| IBIS file 144lqfp.ibs generated by Viper version: 2017.07.25
[IBIS Ver]   5.0
[Comment Char]   |_char
[File Name]   144lqfp.ibs
[File Rev]   1
[Date]   Wed Apr 18 11:55:22 2018
[Source]   Freescale Viper 2017.07.25
[Notes]
[Disclaimer] IMPORTANT NOTICE
  This information is provided on an AS IS basis and without warranty.
  IN NO EVENT SHALL Freescale BE LIABLE FOR INCIDENTAL OR CONSEQUENTIAL
  DAMAGES ARISING FROM USE OF THIS INFORMATION. THIS DISCLAIMER OF
  WARRANTY EXTENDS TO THE USER OF THE INFORMATION, AND TO THEIR CUSTOMERS
  OR USERS OF PRODUCTS  AND IS IN LIEU OF ALL WARRANTIES WHETHER EXPRESS,
  IMPLIED, OR STATUTORY, INCLUDING IMPLIED WARRANTIES OF MERCHANTABILITY
  OR FITNESS FOR PARTICULAR PURPOSE.
  Freescale does not represent or warrant that the information furnished
  hereunder is free of infringement of any third party patents,
  copyrights, trade secrets, or other intellectual property rights.
  Freescale does not represent or warrant that the information is free of
  defect, or that it meets any particular standard, requirements or need
  of the user of the infomation or their customers.
  Freescale reserves the right to change the information in this file
  without notice.
   http://www.freescale.com
[Copyright]   (C) Copyright Freescale 2004 - 2018, All Rights Reserved.
|   144LQFP
[Component]   144LQFP
[Manufacturer]   FREESCALE
[Package]
| variable   typ   min   max
R_pkg   0.23631   0.21255   0.27668
L_pkg   6.725e-09   6.219e-09   7.763e-09
C_pkg   7.045e-13   5.974e-13   8.478e-13
[Pin] signal_name   model_name   R_pin   L_pin   C_pin
1   GPIO_EMC_14   gpio   0.27319   7.763e-09 7.620e-13
2   GPIO_EMC_13   gpio   0.24922   7.284e-09 7.877e-13
3   GPIO_EMC_12   gpio   0.25596   7.201e-09 8.198e-13
4   GPIO_EMC_11   gpio   0.24258   6.690e-09 7.773e-13
5   VDD_SOC_IN   POWER   NA   NA   NA
6   NC   NC   NA   NA   NA
7   GPIO_EMC_10   gpio   0.22716   6.478e-09 7.216e-13
8   GPIO_EMC_09   gpio   0.23253   6.549e-09 7.118e-13
9   GPIO_EMC_08   gpio   0.21792   6.312e-09 7.130e-13
10   GPIO_EMC_07   gpio   0.22722   6.434e-09 6.632e-13
11   NVCC_GPIO   POWER   NA   NA   NA
12   GPIO_EMC_06   gpio   0.21323   6.350e-09 6.818e-13
13   GPIO_EMC_05   gpio   0.2234   6.650e-09 6.747e-13
14   GPIO_EMC_04   gpio   0.22404   6.772e-09 6.509e-13
15   GPIO_EMC_03   gpio   0.21613   6.689e-09 6.468e-13
16   GPIO_EMC_02   gpio   0.22926   6.931e-09 6.556e-13
17   GPIO_EMC_01   gpio   0.22816   6.913e-09 6.110e-13
18   GPIO_EMC_00   gpio   0.26205   7.440e-09 6.211e-13
19   GPIO_SD_B1_11   gpio   0.26047   7.181e-09 6.075e-13
20   NVCC_GPIO   POWER   NA   NA   NA
21   GPIO_SD_B1_10   gpio   0.24307   6.886e-09 6.379e-13
22   GPIO_SD_B1_09   gpio   0.23465   6.862e-09 6.668e-13
23   GPIO_SD_B1_08   gpio   0.22372   6.608e-09 6.606e-13
24   GPIO_SD_B1_07   gpio   0.23361   6.711e-09 6.776e-13
25   GPIO_SD_B1_06   gpio   0.22833   6.612e-09 6.719e-13
26   GPIO_SD_B1_05   gpio   0.24019   6.758e-09 7.358e-13
27   GPIO_SD_B1_04   gpio   0.23557   6.606e-09 7.328e-13
28   GPIO_SD_B1_03   gpio   0.25289   6.532e-09 7.645e-13
29   NVCC_GPIO   POWER   NA   NA   NA
30   GPIO_SD_B1_02   gpio   0.26218   6.601e-09 7.491e-13
31   VDD_SOC_IN   POWER   NA   NA   NA
32   GPIO_SD_B1_01   gpio   0.25369   6.647e-09 8.100e-13
33   GPIO_SD_B1_00   gpio   0.27668   6.878e-09 8.292e-13
34   DCDC_IN   POWER   NA   NA   NA
35   DCDC_GND   GND   NA   NA   NA
36   NC   NC   NA   NA   NA
37   DCDC_PSWITCH   POWER   NA   NA   NA
38   DCDC_IN_Q   POWER   NA   NA   NA
39   VDD_SOC_IN   POWER   NA   NA   NA
40   NC   NC   NA   NA   NA
41   GPIO_SD_B0_06   gpio   0.24784   6.847e-09 7.446e-13
42   GPIO_SD_B0_05   gpio   0.23425   6.606e-09 7.288e-13
43   GPIO_SD_B0_04   gpio   0.23978   6.581e-09 7.445e-13
44   NVCC_SD0   POWER   NA   NA   NA
45   GPIO_SD_B0_03   gpio   0.23499   6.428e-09 7.074e-13
46   GPIO_SD_B0_02   gpio   0.22524   6.518e-09 6.811e-13
47   GPIO_SD_B0_01   gpio   0.21255   6.369e-09 6.751e-13
48   GPIO_SD_B0_00   gpio   0.22018   6.545e-09 6.743e-13
49   ONOFF   gpio   0.22022   6.591e-09 6.545e-13
50   POR_B   gpio   0.22145   6.657e-09 6.500e-13
51   TEST_MODE   gpio   0.21301   6.530e-09 6.305e-13
52   WAKEUP   gpio   0.22627   6.774e-09 6.197e-13
53   PMIC_ON_REQ   gpio   0.22495   6.778e-09 6.119e-13
54   PMIC_STBY_REQ   gpio   0.25873   7.238e-09 6.013e-13
55   VDD_SNVS_IN   POWER   NA   NA   NA
56   VDD_SNVS_CAP   POWER   NA   NA   NA
57   RTC_XTALI   NC   0.23318   6.569e-09 6.200e-13
58   RTC_XTALO   NC   0.22932   6.412e-09 6.458e-13
59   USB_OTG1_VBUS   NC   NA   NA   NA
60   NC   NC   NA   NA   NA
61   VDD_USB_CAP   NC   NA   NA   NA
62   USB_OTG1_DN   NC   0.23049   6.219e-09 6.692e-13
63   USB_OTG1_DP   NC   0.23382   6.238e-09 7.381e-13
64   NGND_KEL0   GND   NA   NA   NA
65   VDD_HIGH_CAP   POWER   NA   NA   NA
66   USB_OTG1_CHD_B   NC   0.23453   6.262e-09 7.522e-13
67   XTALI   NC   0.24304   6.614e-09 7.504e-13
68   XTALO   NC   0.25011   6.724e-09 7.704e-13
69   VDD_HIGH_IN   POWER   NA   NA   NA
70   NC   NC   NA   NA   NA
71   GPANAIO   NC   0.25746   6.958e-09 7.980e-13
72   NVCC_PLL   POWER   NA   NA   NA
73   VDDA_ADC_3P3   POWER   NA   NA   NA
74   GPIO_AD_B1_15   gpio   0.25409   6.952e-09 8.420e-13
75   GPIO_AD_B1_14   gpio   0.25632   6.963e-09 8.478e-13
76   GPIO_AD_B1_13   gpio   0.25252   6.929e-09 7.716e-13
77   NC   NC   NA   NA   NA
78   GPIO_AD_B1_12   gpio   0.24265   6.738e-09 7.369e-13
79   GPIO_AD_B1_11   gpio   0.23034   6.449e-09 7.323e-13
80   GPIO_AD_B1_10   gpio   0.23308   6.558e-09 7.263e-13
81   GPIO_AD_B1_09   gpio   0.22922   6.558e-09 7.224e-13
82   GPIO_AD_B1_08   gpio   0.21958   6.371e-09 7.084e-13
83   GPIO_AD_B1_07   gpio   0.2282   6.393e-09 7.151e-13
84   GPIO_AD_B1_06   gpio   0.23128   6.391e-09 6.709e-13
85   NC   NC   NA   NA   NA
86   VDD_SOC_IN   POWER   NA   NA   NA
87   GPIO_AD_B1_05   gpio   0.22109   6.396e-09 6.938e-13
88   GPIO_AD_B1_04   gpio   0.23176   6.820e-09 6.617e-13
89   GPIO_AD_B1_03   gpio   0.2259   6.807e-09 6.341e-13
90   GPIO_AD_B1_02   gpio   0.2578   7.521e-09 5.976e-13
91   GPIO_AD_B1_01   gpio   0.24916   7.279e-09 5.978e-13
92   GPIO_AD_B1_00   gpio   0.24244   6.931e-09 6.196e-13
93   GPIO_AD_B0_15   gpio   0.23462   6.875e-09 6.702e-13
94   GPIO_AD_B0_14   gpio   0.21942   6.541e-09 6.321e-13
95   GPIO_AD_B0_13   gpio   0.22448   6.708e-09 6.624e-13
96   GPIO_AD_B0_12   gpio   0.22263   6.609e-09 6.816e-13
97   GPIO_AD_B0_11   gpio   0.21559   6.396e-09 6.793e-13
98   GPIO_AD_B0_10   gpio   0.22709   6.461e-09 6.804e-13
99   GPIO_AD_B0_09   gpio   0.22347   6.302e-09 7.026e-13
100   GPIO_AD_B0_08   gpio   0.23203   6.436e-09 7.127e-13
101   GPIO_AD_B0_07   gpio   0.2232   6.229e-09 7.231e-13
102   VDD_SOC_IN   POWER   NA   NA   NA
103   NC   NC   NA   NA   NA
104   NC   NC   NA   NA   NA
105   GPIO_AD_B0_06   gpio   0.23499   6.864e-09 7.362e-13
106   GPIO_AD_B0_05   gpio   0.24648   7.161e-09 8.049e-13
107   GPIO_AD_B0_04   gpio   0.24526   7.309e-09 8.157e-13
108   GPIO_AD_B0_03   gpio   0.26036   7.662e-09 7.794e-13
109   GPIO_AD_B0_02   gpio   0.26315   7.383e-09 7.807e-13
110   GPIO_AD_B0_01   gpio   0.26589   7.252e-09 8.095e-13
111   GPIO_AD_B0_00   gpio   0.26336   6.854e-09 7.971e-13
112   NC   NC   NA   NA   NA
113   NC   NC   NA   NA   NA
114   VDD_SOC_IN   POWER   NA   NA   NA
115   GPIO_EMC_41   gpio   0.22452   6.470e-09 7.317e-13
116   GPIO_EMC_40   gpio   0.23083   6.535e-09 7.263e-13
117   GPIO_EMC_39   gpio   0.22168   6.332e-09 7.381e-13
118   GPIO_EMC_38   gpio   0.23093   6.497e-09 7.401e-13
119   GPIO_EMC_37   gpio   0.23081   6.423e-09 7.303e-13
120   GPIO_EMC_36   gpio   0.22714   6.494e-09 7.167e-13
121   GPIO_EMC_35   gpio   0.21462   6.464e-09 6.823e-13
122   GPIO_EMC_34   gpio   0.22438   6.655e-09 6.932e-13
123   GPIO_EMC_33   gpio   0.21793   6.470e-09 6.273e-13
124   GPIO_EMC_32   gpio   0.23516   6.805e-09 6.307e-13
125   GPIO_EMC_31   gpio   0.24148   6.948e-09 6.305e-13
126   GPIO_EMC_30   gpio   0.25496   7.362e-09 6.088e-13
127   GPIO_EMC_29   gpio   0.2576   7.422e-09 5.974e-13
128   GPIO_EMC_28   gpio   0.24014   7.035e-09 6.374e-13
129   GPIO_EMC_27   gpio   0.22626   6.621e-09 6.383e-13
130   GPIO_EMC_26   gpio   0.23483   6.649e-09 6.554e-13
131   GPIO_EMC_25   gpio   0.23202   6.549e-09 6.551e-13
132   GPIO_EMC_24   gpio   0.22925   6.491e-09 6.599e-13
133   GPIO_EMC_23   gpio   0.2212   6.232e-09 6.790e-13
134   VDD_SOC_IN   POWER   NA   NA   NA
135   NC   NC   NA   NA   NA
136   GPIO_EMC_22   gpio   0.22481   6.353e-09 6.683e-13
137   GPIO_EMC_21   gpio   0.22739   6.524e-09 7.340e-13
138   GPIO_EMC_20   gpio   0.24177   6.765e-09 7.486e-13
139   GPIO_EMC_19   gpio   0.23809   6.755e-09 7.541e-13
140   GPIO_EMC_18   gpio   0.24061   6.892e-09 7.906e-13
141   GPIO_EMC_17   gpio   0.23882   6.883e-09 8.027e-13
142   GPIO_EMC_16   gpio   0.25453   7.072e-09 8.171e-13
143   GPIO_EMC_15   gpio   0.257   7.017e-09 8.337e-13
144   NC   NC   NA   NA   NA
145   NC   NC   NA   NA   NA
[Pin Mapping]   pulldown_ref   pullup_ref
1   NC   NC
2   NC   NC
3   NC   NC
4   NC   NC
5   NC   VDD_SOC_IN
6   NC   NC
7   NC   NC
8   NC   NC
9   NC   NC
10   NC   NC
11   NC   NVCC_GPIO
12   NC   NC
13   NC   NC
14   NC   NC
15   NC   NC
16   NC   NC
17   NC   NC
18   NC   NC
19   NC   NC
20   NC   NVCC_GPIO
21   NC   NC
22   NC   NC
23   NC   NC
24   NC   NC
25   NC   NC
26   NC   NC
27   NC   NC
28   NC   NC
29   NC   NVCC_GPIO
30   NC   NC
31   NC   VDD_SOC_IN
32   NC   NC
33   NC   NC
34   NC   DCDC_IN
35   DCDC_GND   NC
36   NC   NC
37   NC   DCDC_PSWITCH
38   NC   DCDC_IN_Q
39   NC   VDD_SOC_IN
40   NC   NC
41   NC   NC
42   NC   NC
43   NC   NC
44   NC   NVCC_SD0
45   NC   NC
46   NC   NC
47   NC   NC
48   NC   NC
49   NC   NC
50   NC   NC
51   NC   NC
52   NC   NC
53   NC   NC
54   NC   NC
55   NC   VDD_SNVS_IN
56   NC   VDD_SNVS_CAP
57   NC   NC
58   NC   NC
59   NC   NC
60   NC   NC
61   NC   NC
62   NC   NC
63   NC   NC
64   NGND_KEL0   NC
65   NC   VDD_HIGH_CAP
66   NC   NC
67   NC   NC
68   NC   NC
69   NC   VDD_HIGH_IN
70   NC   NC
71   NC   NC
72   NC   NVCC_PLL
73   NC   VDDA_ADC_3P3
74   NC   NC
75   NC   NC
76   NC   NC
77   NC   NC
78   NC   NC
79   NC   NC
80   NC   NC
81   NC   NC
82   NC   NC
83   NC   NC
84   NC   NC
85   NC   NC
86   NC   VDD_SOC_IN
87   NC   NC
88   NC   NC
89   NC   NC
90   NC   NC
91   NC   NC
92   NC   NC
93   NC   NC
94   NC   NC
95   NC   NC
96   NC   NC
97   NC   NC
98   NC   NC
99   NC   NC
100   NC   NC
101   NC   NC
102   NC   VDD_SOC_IN
103   NC   NC
104   NC   NC
105   NC   NC
106   NC   NC
107   NC   NC
108   NC   NC
109   NC   NC
110   NC   NC
111   NC   NC
112   NC   NC
113   NC   NC
114   NC   VDD_SOC_IN
115   NC   NC
116   NC   NC
117   NC   NC
118   NC   NC
119   NC   NC
120   NC   NC
121   NC   NC
122   NC   NC
123   NC   NC
124   NC   NC
125   NC   NC
126   NC   NC
127   NC   NC
128   NC   NC
129   NC   NC
130   NC   NC
131   NC   NC
132   NC   NC
133   NC   NC
134   NC   VDD_SOC_IN
135   NC   NC
136   NC   NC
137   NC   NC
138   NC   NC
139   NC   NC
140   NC   NC
141   NC   NC
142   NC   NC
143   NC   NC
144   NC   NC
145   NC   NC
|*   Model Selector   *
[Model Selector] gpio
gpio1p8_ds111_sr111_mio   GPIO, 1.8V,extra drive,fast sr,max fsel
gpio1p8_ds111_sr110_mio   GPIO, 1.8V,extra drive,fast sr,fast fsel
gpio1p8_ds111_sr101_mio   GPIO, 1.8V,extra drive,fast sr,medium fsel
gpio1p8_ds111_sr100_mio   GPIO, 1.8V,extra drive,fast sr,slow fsel
gpio1p8_ds111_sr011_mio   GPIO, 1.8V,extra drive,slow sr,max fsel
gpio1p8_ds111_sr010_mio   GPIO, 1.8V,extra drive,slow sr,fast fsel
gpio1p8_ds111_sr001_mio   GPIO, 1.8V,extra drive,slow sr,medium fsel
gpio1p8_ds111_sr000_mio   GPIO, 1.8V,extra drive,slow sr,slow fsel
gpio1p8_ds110_sr111_mio   GPIO, 1.8V,extra drive,fast sr,max fsel
gpio1p8_ds110_sr110_mio   GPIO, 1.8V,extra drive,fast sr,fast fsel
gpio1p8_ds110_sr101_mio   GPIO, 1.8V,extra drive,fast sr,medium fsel
gpio1p8_ds110_sr100_mio   GPIO, 1.8V,extra drive,fast sr,slow fsel
gpio1p8_ds110_sr011_mio   GPIO, 1.8V,extra drive,slow sr,max fsel
gpio1p8_ds110_sr010_mio   GPIO, 1.8V,extra drive,slow sr,fast fsel
gpio1p8_ds110_sr001_mio   GPIO, 1.8V,extra drive,slow sr,medium fsel
gpio1p8_ds110_sr000_mio   GPIO, 1.8V,extra drive,slow sr,slow fsel
gpio1p8_ds101_sr111_mio   GPIO, 1.8V,max drive,fast sr,max fsel
gpio1p8_ds101_sr110_mio   GPIO, 1.8V,max drive,fast sr,fast fsel
gpio1p8_ds101_sr101_mio   GPIO, 1.8V,max drive,fast sr,medium fsel
gpio1p8_ds101_sr100_mio   GPIO, 1.8V,max drive,fast sr,slow fsel
gpio1p8_ds101_sr011_mio   GPIO, 1.8V,max drive,slow sr,max fsel
gpio1p8_ds101_sr010_mio   GPIO, 1.8V,max drive,slow sr,fast fsel
gpio1p8_ds101_sr001_mio   GPIO, 1.8V,max drive,slow sr,medium fsel
gpio1p8_ds101_sr000_mio   GPIO, 1.8V,max drive,slow sr,slow fsel
gpio1p8_ds100_sr111_mio   GPIO, 1.8V,extra drive,fast sr,max fsel
gpio1p8_ds100_sr110_mio   GPIO, 1.8V,extra drive,fast sr,fast fsel
gpio1p8_ds100_sr101_mio   GPIO, 1.8V,extra drive,fast sr,medium fsel
gpio1p8_ds100_sr100_mio   GPIO, 1.8V,extra drive,fast sr,slow fsel
gpio1p8_ds100_sr011_mio   GPIO, 1.8V,extra drive,slow sr,max fsel
gpio1p8_ds100_sr010_mio   GPIO, 1.8V,extra drive,slow sr,fast fsel
gpio1p8_ds100_sr001_mio   GPIO, 1.8V,extra drive,slow sr,medium fsel
gpio1p8_ds100_sr000_mio   GPIO, 1.8V,extra drive,slow sr,slow fsel
gpio1p8_ds011_sr111_mio   GPIO, 1.8V,high drive,fast sr,max fsel
gpio1p8_ds011_sr110_mio   GPIO, 1.8V,high drive,fast sr,fast fsel
gpio1p8_ds011_sr101_mio   GPIO, 1.8V,high drive,fast sr,medium fsel
gpio1p8_ds011_sr100_mio   GPIO, 1.8V,high drive,fast sr,slow fsel
gpio1p8_ds011_sr011_mio   GPIO, 1.8V,high drive,slow sr,max fsel
gpio1p8_ds011_sr010_mio   GPIO, 1.8V,high drive,slow sr,fast fsel
gpio1p8_ds011_sr001_mio   GPIO, 1.8V,high drive,slow sr,medium fsel
gpio1p8_ds011_sr000_mio   GPIO, 1.8V,high drive,slow sr,slow fsel
gpio1p8_ds010_sr111_mio   GPIO, 1.8V,medium drive,fast sr,max fsel
gpio1p8_ds010_sr110_mio   GPIO, 1.8V,medium drive,fast sr,fast fsel
gpio1p8_ds010_sr101_mio   GPIO, 1.8V,medium drive,fast sr,medium fsel
gpio1p8_ds010_sr100_mio   GPIO, 1.8V,medium drive,fast sr,slow fsel
gpio1p8_ds010_sr011_mio   GPIO, 1.8V,medium drive,slow sr,max fsel
gpio1p8_ds010_sr010_mio   GPIO, 1.8V,medium drive,slow sr,fast fsel
gpio1p8_ds010_sr001_mio   GPIO, 1.8V,medium drive,slow sr,medium fsel
gpio1p8_ds010_sr000_mio   GPIO, 1.8V,medium drive,slow sr,slow fsel
gpio1p8_ds001_sr111_mio   GPIO, 1.8V,low drive,fast sr,max fsel
gpio1p8_ds001_sr110_mio   GPIO, 1.8V,low drive,fast sr,fast fsel
gpio1p8_ds001_sr101_mio   GPIO, 1.8V,low drive,fast sr,medium fsel
gpio1p8_ds001_sr100_mio   GPIO, 1.8V,low drive,fast sr,slow fsel
gpio1p8_ds001_sr011_mio   GPIO, 1.8V,low drive,slow sr,max fsel
gpio1p8_ds001_sr010_mio   GPIO, 1.8V,low drive,slow sr,fast fsel
gpio1p8_ds001_sr001_mio   GPIO, 1.8V,low drive,slow sr,medium fsel
gpio1p8_ds001_sr000_mio   GPIO, 1.8V,low drive,slow sr,slow fsel
gpio2p5_ds111_sr111_mio   GPIO, 2.5V,extra drive,fast sr,max fsel
gpio2p5_ds111_sr110_mio   GPIO, 2.5V,extra drive,fast sr,fast fsel
gpio2p5_ds111_sr101_mio   GPIO, 2.5V,extra drive,fast sr,medium fsel
gpio2p5_ds111_sr100_mio   GPIO, 2.5V,extra drive,fast sr,slow fsel
gpio2p5_ds111_sr011_mio   GPIO, 2.5V,extra drive,slow sr,max fsel
gpio2p5_ds111_sr010_mio   GPIO, 2.5V,extra drive,slow sr,fast fsel
gpio2p5_ds111_sr001_mio   GPIO, 2.5V,extra drive,slow sr,medium fsel
gpio2p5_ds111_sr000_mio   GPIO, 2.5V,extra drive,slow sr,slow fsel
gpio2p5_ds110_sr111_mio   GPIO, 2.5V,extra drive,fast sr,max fsel
gpio2p5_ds110_sr110_mio   GPIO, 2.5V,extra drive,fast sr,fast fsel
gpio2p5_ds110_sr101_mio   GPIO, 2.5V,extra drive,fast sr,medium fsel
gpio2p5_ds110_sr100_mio   GPIO, 2.5V,extra drive,fast sr,slow fsel
gpio2p5_ds110_sr011_mio   GPIO, 2.5V,extra drive,slow sr,max fsel
gpio2p5_ds110_sr010_mio   GPIO, 2.5V,extra drive,slow sr,fast fsel
gpio2p5_ds110_sr001_mio   GPIO, 2.5V,extra drive,slow sr,medium fsel
gpio2p5_ds110_sr000_mio   GPIO, 2.5V,extra drive,slow sr,slow fsel
gpio2p5_ds101_sr111_mio   GPIO, 2.5V,max drive,fast sr,max fsel
gpio2p5_ds101_sr110_mio   GPIO, 2.5V,max drive,fast sr,fast fsel
gpio2p5_ds101_sr101_mio   GPIO, 2.5V,max drive,fast sr,medium fsel
gpio2p5_ds101_sr100_mio   GPIO, 2.5V,max drive,fast sr,slow fsel
gpio2p5_ds101_sr011_mio   GPIO, 2.5V,max drive,slow sr,max fsel
gpio2p5_ds101_sr010_mio   GPIO, 2.5V,max drive,slow sr,fast fsel
gpio2p5_ds101_sr001_mio   GPIO, 2.5V,max drive,slow sr,medium fsel
gpio2p5_ds101_sr000_mio   GPIO, 2.5V,max drive,slow sr,slow fsel
gpio2p5_ds100_sr111_mio   GPIO, 2.5V,extra drive,fast sr,max fsel
gpio2p5_ds100_sr110_mio   GPIO, 2.5V,extra drive,fast sr,fast fsel
gpio2p5_ds100_sr101_mio   GPIO, 2.5V,extra drive,fast sr,medium fsel
gpio2p5_ds100_sr100_mio   GPIO, 2.5V,extra drive,fast sr,slow fsel
gpio2p5_ds100_sr011_mio   GPIO, 2.5V,extra drive,slow sr,max fsel
gpio2p5_ds100_sr010_mio   GPIO, 2.5V,extra drive,slow sr,fast fsel
gpio2p5_ds100_sr001_mio   GPIO, 2.5V,extra drive,slow sr,medium fsel
gpio2p5_ds100_sr000_mio   GPIO, 2.5V,extra drive,slow sr,slow fsel
gpio2p5_ds011_sr111_mio   GPIO, 2.5V,high drive,fast sr,max fsel
gpio2p5_ds011_sr110_mio   GPIO, 2.5V,high drive,fast sr,fast fsel
gpio2p5_ds011_sr101_mio   GPIO, 2.5V,high drive,fast sr,medium fsel
gpio2p5_ds011_sr100_mio   GPIO, 2.5V,high drive,fast sr,slow fsel
gpio2p5_ds011_sr011_mio   GPIO, 2.5V,high drive,slow sr,max fsel
gpio2p5_ds011_sr010_mio   GPIO, 2.5V,high drive,slow sr,fast fsel
gpio2p5_ds011_sr001_mio   GPIO, 2.5V,high drive,slow sr,medium fsel
gpio2p5_ds011_sr000_mio   GPIO, 2.5V,high drive,slow sr,slow fsel
gpio2p5_ds010_sr111_mio   GPIO, 2.5V,medium drive,fast sr,max fsel
gpio2p5_ds010_sr110_mio   GPIO, 2.5V,medium drive,fast sr,fast fsel
gpio2p5_ds010_sr101_mio   GPIO, 2.5V,medium drive,fast sr,medium fsel
gpio2p5_ds010_sr100_mio   GPIO, 2.5V,medium drive,fast sr,slow fsel
gpio2p5_ds010_sr011_mio   GPIO, 2.5V,medium drive,slow sr,max fsel
gpio2p5_ds010_sr010_mio   GPIO, 2.5V,medium drive,slow sr,fast fsel
gpio2p5_ds010_sr001_mio   GPIO, 2.5V,medium drive,slow sr,medium fsel
gpio2p5_ds010_sr000_mio   GPIO, 2.5V,medium drive,slow sr,slow fsel
gpio2p5_ds001_sr111_mio   GPIO, 2.5V,low drive,fast sr,max fsel
gpio2p5_ds001_sr110_mio   GPIO, 2.5V,low drive,fast sr,fast fsel
gpio2p5_ds001_sr101_mio   GPIO, 2.5V,low drive,fast sr,medium fsel
gpio2p5_ds001_sr100_mio   GPIO, 2.5V,low drive,fast sr,slow fsel
gpio2p5_ds001_sr011_mio   GPIO, 2.5V,low drive,slow sr,max fsel
gpio2p5_ds001_sr010_mio   GPIO, 2.5V,low drive,slow sr,fast fsel
gpio2p5_ds001_sr001_mio   GPIO, 2.5V,low drive,slow sr,medium fsel
gpio2p5_ds001_sr000_mio   GPIO, 2.5V,low drive,slow sr,slow fsel
gpio3p3_ds111_sr111_mio   GPIO, 3.3V,extra drive,fast sr,max fsel
gpio3p3_ds111_sr110_mio   GPIO, 3.3V,extra drive,fast sr,fast fsel
gpio3p3_ds111_sr101_mio   GPIO, 3.3V,extra drive,fast sr,medium fsel
gpio3p3_ds111_sr100_mio   GPIO, 3.3V,extra drive,fast sr,slow fsel
gpio3p3_ds111_sr011_mio   GPIO, 3.3V,extra drive,slow sr,max fsel
gpio3p3_ds111_sr010_mio   GPIO, 3.3V,extra drive,slow sr,fast fsel
gpio3p3_ds111_sr001_mio   GPIO, 3.3V,extra drive,slow sr,medium fsel
gpio3p3_ds111_sr000_mio   GPIO, 3.3V,extra drive,slow sr,slow fsel
gpio3p3_ds110_sr111_mio   GPIO, 3.3V,extra drive,fast sr,max fsel
gpio3p3_ds110_sr110_mio   GPIO, 3.3V,extra drive,fast sr,fast fsel
gpio3p3_ds110_sr101_mio   GPIO, 3.3V,extra drive,fast sr,medium fsel
gpio3p3_ds110_sr100_mio   GPIO, 3.3V,extra drive,fast sr,slow fsel
gpio3p3_ds110_sr011_mio   GPIO, 3.3V,extra drive,slow sr,max fsel
gpio3p3_ds110_sr010_mio   GPIO, 3.3V,extra drive,slow sr,fast fsel
gpio3p3_ds110_sr001_mio   GPIO, 3.3V,extra drive,slow sr,medium fsel
gpio3p3_ds110_sr000_mio   GPIO, 3.3V,extra drive,slow sr,slow fsel
gpio3p3_ds101_sr111_mio   GPIO, 3.3V,max drive,fast sr,max fsel
gpio3p3_ds101_sr110_mio   GPIO, 3.3V,max drive,fast sr,fast fsel
gpio3p3_ds101_sr101_mio   GPIO, 3.3V,max drive,fast sr,medium fsel
gpio3p3_ds101_sr100_mio   GPIO, 3.3V,max drive,fast sr,slow fsel
gpio3p3_ds101_sr011_mio   GPIO, 3.3V,max drive,slow sr,max fsel
gpio3p3_ds101_sr010_mio   GPIO, 3.3V,max drive,slow sr,fast fsel
gpio3p3_ds101_sr001_mio   GPIO, 3.3V,max drive,slow sr,medium fsel
gpio3p3_ds101_sr000_mio   GPIO, 3.3V,max drive,slow sr,slow fsel
gpio3p3_ds100_sr111_mio   GPIO, 3.3V,extra drive,fast sr,max fsel
gpio3p3_ds100_sr110_mio   GPIO, 3.3V,extra drive,fast sr,fast fsel
gpio3p3_ds100_sr101_mio   GPIO, 3.3V,extra drive,fast sr,medium fsel
gpio3p3_ds100_sr100_mio   GPIO, 3.3V,extra drive,fast sr,slow fsel
gpio3p3_ds100_sr011_mio   GPIO, 3.3V,extra drive,slow sr,max fsel
gpio3p3_ds100_sr010_mio   GPIO, 3.3V,extra drive,slow sr,fast fsel
gpio3p3_ds100_sr001_mio   GPIO, 3.3V,extra drive,slow sr,medium fsel
gpio3p3_ds100_sr000_mio   GPIO, 3.3V,extra drive,slow sr,slow fsel
gpio3p3_ds011_sr111_mio   GPIO, 3.3V,high drive,fast sr,max fsel
gpio3p3_ds011_sr110_mio   GPIO, 3.3V,high drive,fast sr,fast fsel
gpio3p3_ds011_sr101_mio   GPIO, 3.3V,high drive,fast sr,medium fsel
gpio3p3_ds011_sr100_mio   GPIO, 3.3V,high drive,fast sr,slow fsel
gpio3p3_ds011_sr011_mio   GPIO, 3.3V,high drive,slow sr,max fsel
gpio3p3_ds011_sr010_mio   GPIO, 3.3V,high drive,slow sr,fast fsel
gpio3p3_ds011_sr001_mio   GPIO, 3.3V,high drive,slow sr,medium fsel
gpio3p3_ds011_sr000_mio   GPIO, 3.3V,high drive,slow sr,slow fsel
gpio3p3_ds010_sr111_mio   GPIO, 3.3V,medium drive,fast sr,max fsel
gpio3p3_ds010_sr110_mio   GPIO, 3.3V,medium drive,fast sr,fast fsel
gpio3p3_ds010_sr101_mio   GPIO, 3.3V,medium drive,fast sr,medium fsel
gpio3p3_ds010_sr100_mio   GPIO, 3.3V,medium drive,fast sr,slow fsel
gpio3p3_ds010_sr011_mio   GPIO, 3.3V,medium drive,slow sr,max fsel
gpio3p3_ds010_sr010_mio   GPIO, 3.3V,medium drive,slow sr,fast fsel
gpio3p3_ds010_sr001_mio   GPIO, 3.3V,medium drive,slow sr,medium fsel
gpio3p3_ds010_sr000_mio   GPIO, 3.3V,medium drive,slow sr,slow fsel
gpio3p3_ds001_sr111_mio   GPIO, 3.3V,low drive,fast sr,max fsel
gpio3p3_ds001_sr110_mio   GPIO, 3.3V,low drive,fast sr,fast fsel
gpio3p3_ds001_sr101_mio   GPIO, 3.3V,low drive,fast sr,medium fsel
gpio3p3_ds001_sr100_mio   GPIO, 3.3V,low drive,fast sr,slow fsel
gpio3p3_ds001_sr011_mio   GPIO, 3.3V,low drive,slow sr,max fsel
gpio3p3_ds001_sr010_mio   GPIO, 3.3V,low drive,slow sr,fast fsel
gpio3p3_ds001_sr001_mio   GPIO, 3.3V,low drive,slow sr,medium fsel
gpio3p3_ds001_sr000_mio   GPIO, 3.3V,low drive,slow sr,slow fsel
| End [Component] 144LQFP
| Models and submodels in the file (168): gpio1p8_ds001_sr000_mio (I/O), gpio1p8_ds001_sr001_mio (I/O), gpio1p8_ds001_sr010_mio (I/O), gpio1p8_ds001_sr011_mio (I/O), gpio1p8_ds001_sr100_mio (I/O), gpio1p8_ds001_sr101_mio (I/O), gpio1p8_ds001_sr110_mio (I/O), gpio1p8_ds001_sr111_mio (I/O), gpio1p8_ds010_sr000_mio (I/O), gpio1p8_ds010_sr001_mio (I/O), gpio1p8_ds010_sr010_mio (I/O), gpio1p8_ds010_sr011_mio (I/O), gpio1p8_ds010_sr100_mio (I/O), gpio1p8_ds010_sr101_mio (I/O), gpio1p8_ds010_sr110_mio (I/O), gpio1p8_ds010_sr111_mio (I/O), gpio1p8_ds011_sr000_mio (I/O), gpio1p8_ds011_sr001_mio (I/O), gpio1p8_ds011_sr010_mio (I/O), gpio1p8_ds011_sr011_mio (I/O), gpio1p8_ds011_sr100_mio (I/O), gpio1p8_ds011_sr101_mio (I/O), gpio1p8_ds011_sr110_mio (I/O), gpio1p8_ds011_sr111_mio (I/O), gpio1p8_ds100_sr000_mio (I/O), gpio1p8_ds100_sr001_mio (I/O), gpio1p8_ds100_sr010_mio (I/O), gpio1p8_ds100_sr011_mio (I/O), gpio1p8_ds100_sr100_mio (I/O), gpio1p8_ds100_sr101_mio (I/O), gpio1p8_ds100_sr110_mio (I/O), gpio1p8_ds100_sr111_mio (I/O), gpio1p8_ds101_sr000_mio (I/O), gpio1p8_ds101_sr001_mio (I/O), gpio1p8_ds101_sr010_mio (I/O), gpio1p8_ds101_sr011_mio (I/O), gpio1p8_ds101_sr100_mio (I/O), gpio1p8_ds101_sr101_mio (I/O), gpio1p8_ds101_sr110_mio (I/O), gpio1p8_ds101_sr111_mio (I/O), gpio1p8_ds110_sr000_mio (I/O), gpio1p8_ds110_sr001_mio (I/O), gpio1p8_ds110_sr010_mio (I/O), gpio1p8_ds110_sr011_mio (I/O), gpio1p8_ds110_sr100_mio (I/O), gpio1p8_ds110_sr101_mio (I/O), gpio1p8_ds110_sr110_mio (I/O), gpio1p8_ds110_sr111_mio (I/O), gpio1p8_ds111_sr000_mio (I/O), gpio1p8_ds111_sr001_mio (I/O), gpio1p8_ds111_sr010_mio (I/O), gpio1p8_ds111_sr011_mio (I/O), gpio1p8_ds111_sr100_mio (I/O), gpio1p8_ds111_sr101_mio (I/O), gpio1p8_ds111_sr110_mio (I/O), gpio1p8_ds111_sr111_mio (I/O), gpio2p5_ds001_sr000_mio (I/O), gpio2p5_ds001_sr001_mio (I/O), gpio2p5_ds001_sr010_mio (I/O), gpio2p5_ds001_sr011_mio (I/O), gpio2p5_ds001_sr100_mio (I/O), gpio2p5_ds001_sr101_mio (I/O), gpio2p5_ds001_sr110_mio (I/O), gpio2p5_ds001_sr111_mio (I/O), gpio2p5_ds010_sr000_mio (I/O), gpio2p5_ds010_sr001_mio (I/O), gpio2p5_ds010_sr010_mio (I/O), gpio2p5_ds010_sr011_mio (I/O), gpio2p5_ds010_sr100_mio (I/O), gpio2p5_ds010_sr101_mio (I/O), gpio2p5_ds010_sr110_mio (I/O), gpio2p5_ds010_sr111_mio (I/O), gpio2p5_ds011_sr000_mio (I/O), gpio2p5_ds011_sr001_mio (I/O), gpio2p5_ds011_sr010_mio (I/O), gpio2p5_ds011_sr011_mio (I/O), gpio2p5_ds011_sr100_mio (I/O), gpio2p5_ds011_sr101_mio (I/O), gpio2p5_ds011_sr110_mio (I/O), gpio2p5_ds011_sr111_mio (I/O)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
